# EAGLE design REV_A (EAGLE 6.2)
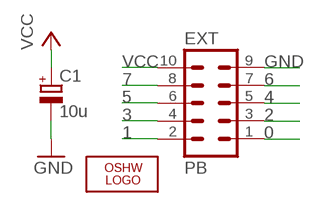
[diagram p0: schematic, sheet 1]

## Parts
C1  10u  CPOL-EUSMCA  [SMC_A]
EXT  PB  ML10  [ML10]
LOGO1  OSHW_LOGO_8MIL  [OSHW_8X150_NOTEXT_MASK]

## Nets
0: EXT.1
1: EXT.2
2: EXT.3
3: EXT.4
4: EXT.5
5: EXT.6
6: EXT.7
7: EXT.8
GND: C1.- EXT.9
VCC: C1.+ EXT.10

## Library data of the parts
C1 = rcl:CPOL-EU: POLARIZED CAPACITOR, European symbol
EXT = con-harting-ml2:ML10: HARTING; OC_FARNELL: unknown; OC_NEWARK: unknown
LOGO1 = ohw-logo:OSHW_LOGO_8MIL

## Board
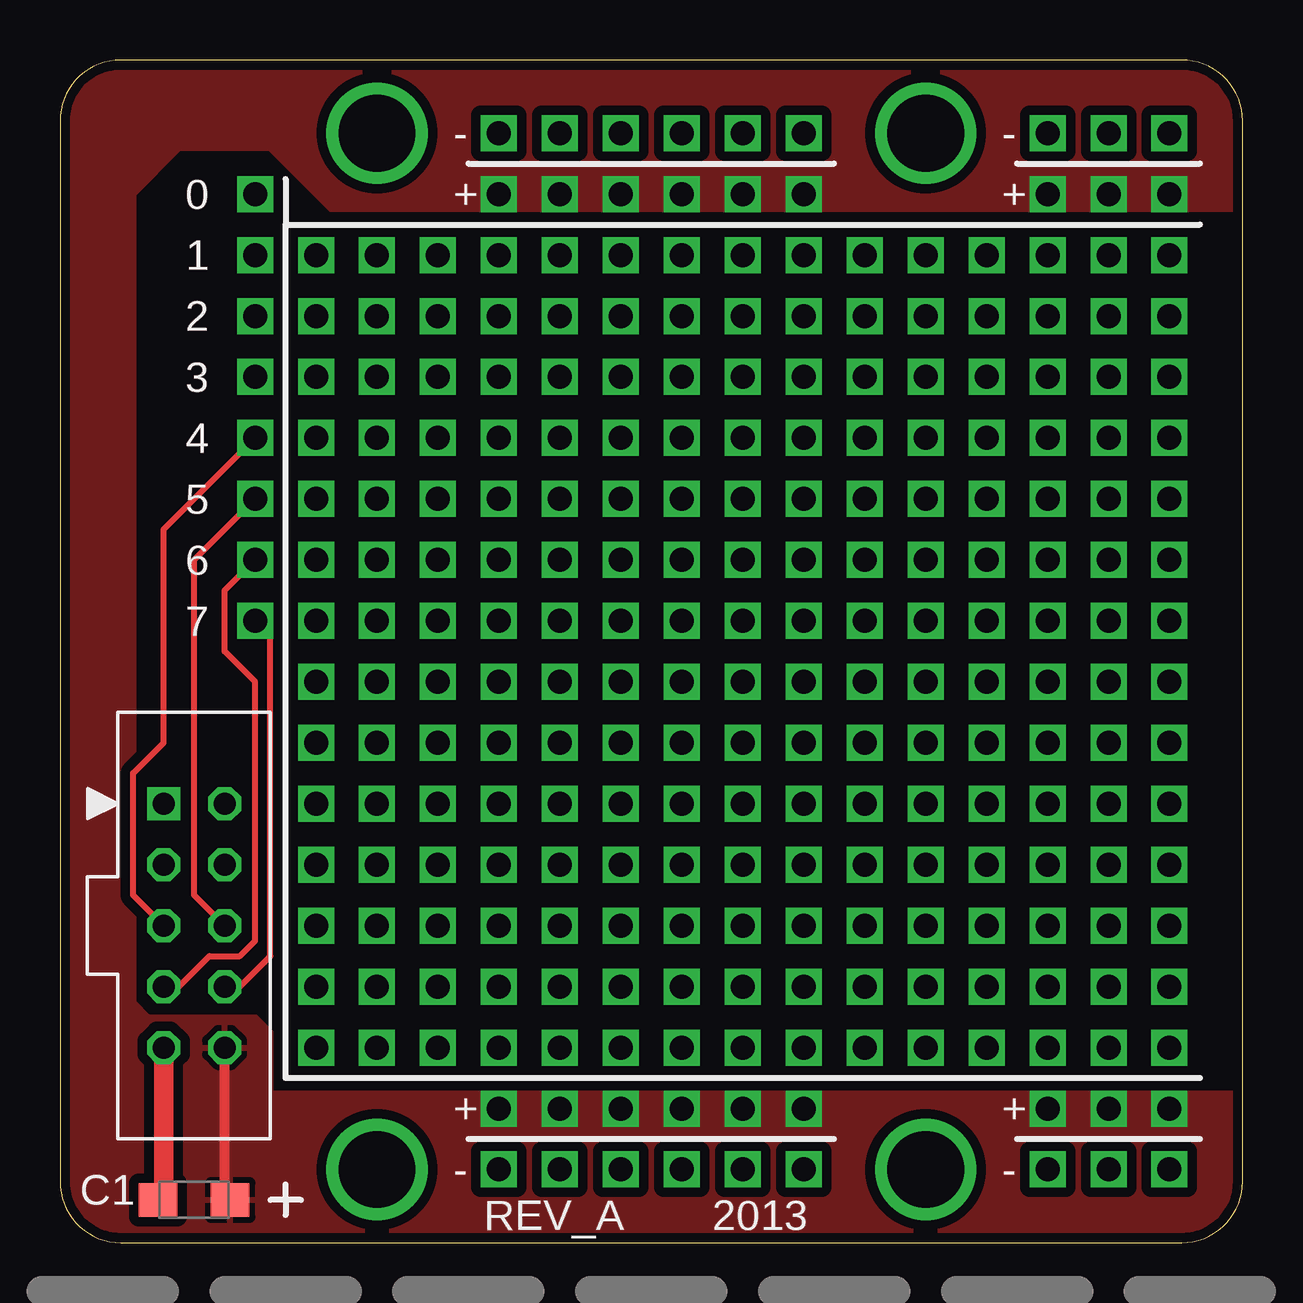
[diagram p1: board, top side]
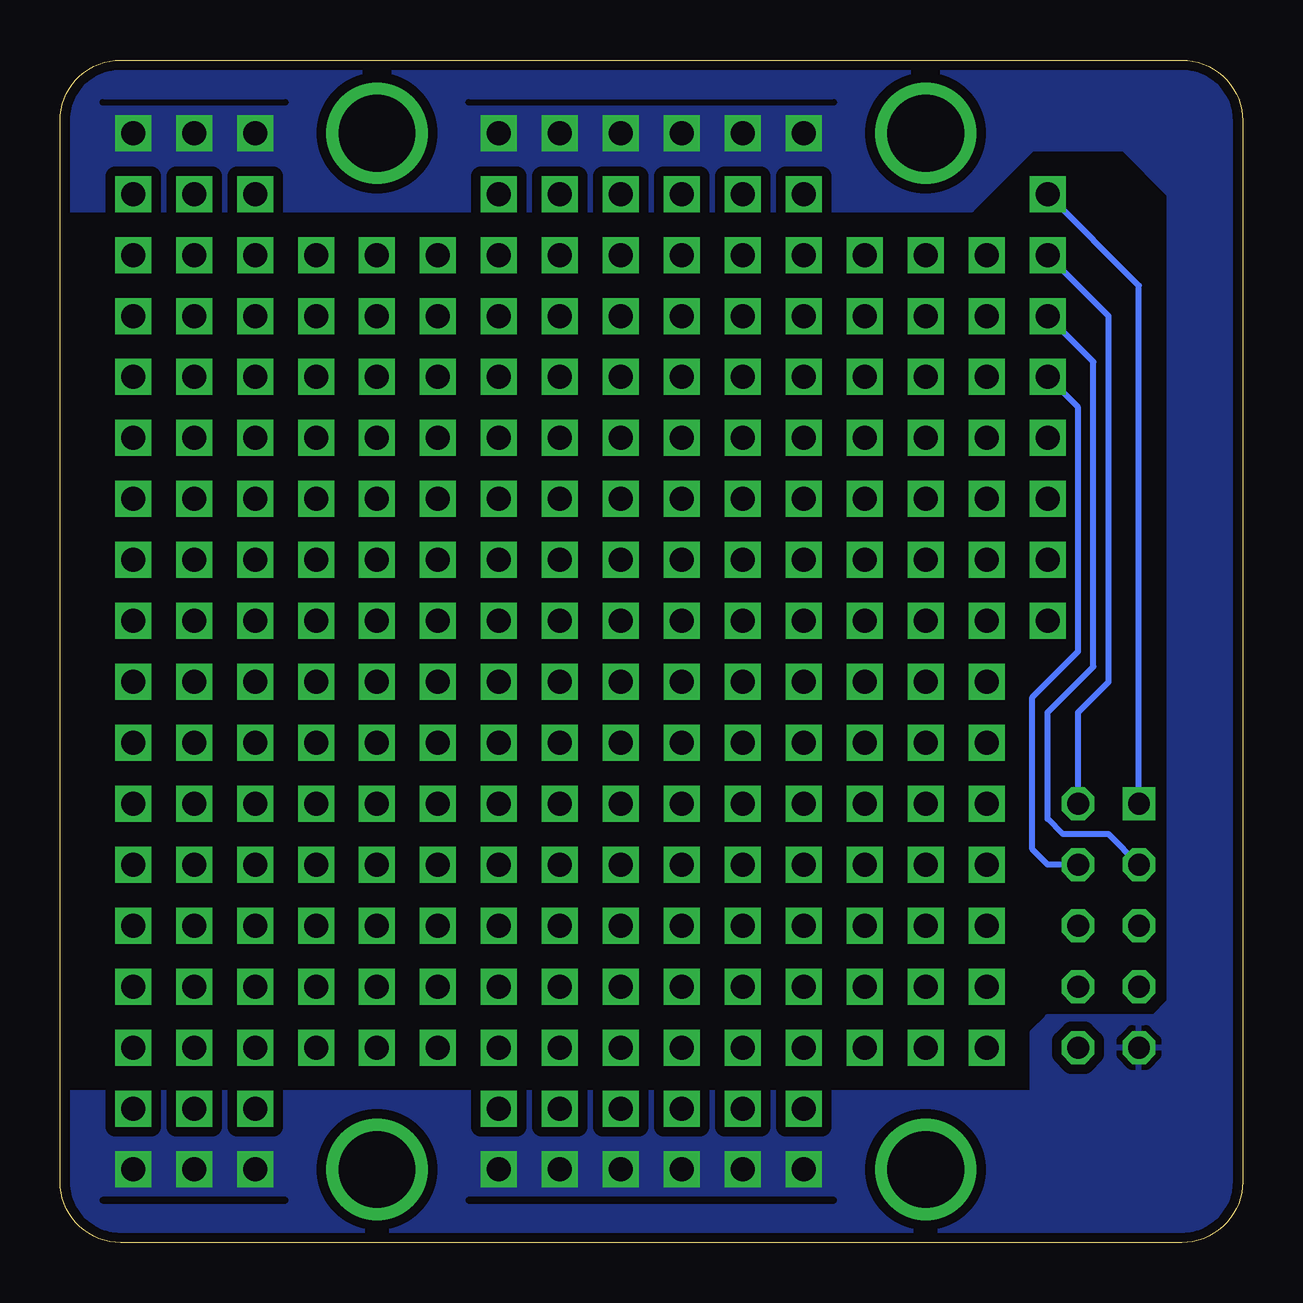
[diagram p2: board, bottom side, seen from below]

Size 49.28 x 49.28 mm. Coordinates in mm from the lower left corner, seen from the top.
Outline: 46.74,49.28 2.54,49.28 arc90 0,46.74 0,2.54 arc90 2.54,0 46.74,0 arc90 49.28,2.54 49.28,46.74 arc90 46.74,49.28
Copper layers (1*2*15*16): Top 0.035mm / dielectric 0.2mm / layer 2 0.0175mm / dielectric 1.1mm / layer 15 0.0175mm / dielectric 0.2mm / Bottom 0.035mm
Design rules: minimum track width 6mil, minimum drill 12mil, track to track 6mil, track to pad 6mil, pad to pad 6mil, via to via 6mil, smd to smd 0mil, copper to edge 10mil, drill to drill 10mil, minimum pad ring 6mil, minimum via ring 6mil, stop-mask expansion 2mil, vias tented up to drill 25mil, thermal gap 10mil

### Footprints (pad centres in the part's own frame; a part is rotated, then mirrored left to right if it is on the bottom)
SMC_A = smd 1.6 x 1.4: + -1.5,0; - 1.5,0
ML10 = drill 0.914 square: 1 -5.08,-1.27 | drill 0.914 octagon: 2 -5.08,1.27; 3 -2.54,-1.27; 4 -2.54,1.27; 5 0,-1.27; 6 0,1.27; 7 2.54,-1.27; 8 2.54,1.27; 9 5.08,-1.27; 10 5.08,1.27

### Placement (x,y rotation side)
C1  5.59,1.78 180 top
EXT  5.59,13.21 270 top
LOGO1  5.59,46.86 315 bottom

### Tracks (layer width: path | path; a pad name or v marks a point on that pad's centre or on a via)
0  (via drill 1)
  Bottom 0.254: EXT.1 4.32,39.88 v8.13,43.69
1  (via drill 1)
  Bottom 0.254: EXT.2 6.86,22.1 5.59,23.37 5.59,38.61 v8.13,41.15
2  (via drill 1)
  Bottom 0.254: EXT.3 5.59,17.02 7.49,17.02 8.13,17.65 8.13,22.1 6.22,24 6.22,36.7 v8.13,38.61
3  (via drill 1)
  Bottom 0.254: v8.13,36.07 6.86,34.8 6.86,24.64 8.76,22.73 8.76,16.38 8.13,15.75 EXT.4
4  (via drill 1)
  Top 0.254: EXT.5 3.05,14.48 3.05,19.56 4.32,20.83 4.32,29.72 v8.13,33.53
5  (via drill 1)
  Top 0.254: EXT.6 5.59,14.48 5.59,28.45 v8.13,30.99
6  (via drill 1)
  Top 0.254: EXT.7 4.95,10.67 6.22,11.94 7.49,11.94 8.13,12.57 8.13,23.37 6.86,24.64 6.86,27.18 v8.13,28.45
7  (via drill 1)
  Top 0.254: EXT.8 7.49,10.67 8.76,11.94 8.76,25.27 v8.13,25.91
GND  (via drill 1)
  Top 0.406: C1.- 4.32,1.78
  Top 0.813: 4.32,1.78 EXT.9
  other vias: 18.29,3.05 20.83,3.05 23.37,3.05 25.91,3.05 28.45,3.05 30.99,3.05 41.15,3.05 43.69,3.05 46.23,3.05 18.29,46.23 20.83,46.23 23.37,46.23 25.91,46.23 28.45,46.23 30.99,46.23 41.15,46.23 43.69,46.23 46.23,46.23
  pour Bottom (isolate 0.406): 50.04,6.22 50.04,-0.76 -0.76,-0.76 -0.76,49.4 47.5,49.4 50.04,46.86 50.04,43.05 11.3,43.05 8.76,45.59 4.95,45.59 3.05,43.69 3.05,10.03 3.68,9.4 8.13,9.4 8.76,8.76 8.76,6.22
N$3  (via drill 3.2)
  other vias: 13.21,46.23
N$4  (via drill 1)
  other vias: 10.67,41.15
N$5  (via drill 1)
  other vias: 13.21,41.15
N$6  (via drill 1)
  other vias: 15.75,41.15
N$7  (via drill 1)
  other vias: 18.29,41.15
N$8  (via drill 1)
  other vias: 20.83,41.15
N$9  (via drill 1)
  other vias: 23.37,41.15
N$10  (via drill 1)
  other vias: 25.91,41.15
N$11  (via drill 1)
  other vias: 28.45,41.15
N$12  (via drill 1)
  other vias: 30.99,41.15
N$13  (via drill 1)
  other vias: 33.53,41.15
N$14  (via drill 1)
  other vias: 36.07,41.15
N$15  (via drill 1)
  other vias: 38.61,41.15
N$16  (via drill 1)
  other vias: 41.15,41.15
N$17  (via drill 1)
  other vias: 43.69,41.15
N$18  (via drill 1)
  other vias: 46.23,41.15
N$21  (via drill 3.2)
  other vias: 36.07,46.23
N$22  (via drill 1)
  other vias: 10.67,38.61
N$23  (via drill 1)
  other vias: 13.21,38.61
N$24  (via drill 1)
  other vias: 15.75,38.61
N$25  (via drill 1)
  other vias: 18.29,38.61
N$26  (via drill 1)
  other vias: 20.83,38.61
N$27  (via drill 1)
  other vias: 23.37,38.61
N$28  (via drill 1)
  other vias: 25.91,38.61
N$29  (via drill 1)
  other vias: 28.45,38.61
N$30  (via drill 1)
  other vias: 30.99,38.61
N$31  (via drill 1)
  other vias: 33.53,38.61
N$32  (via drill 1)
  other vias: 36.07,38.61
N$33  (via drill 1)
  other vias: 38.61,38.61
N$34  (via drill 1)
  other vias: 41.15,38.61
N$35  (via drill 1)
  other vias: 43.69,38.61
N$36  (via drill 1)
  other vias: 46.23,38.61
N$39
  cutout Bottom: 17.02,1.78 32.26,1.78 32.26,1.75 17.02,1.75
N$40  (via drill 1)
  other vias: 10.67,36.07
N$41  (via drill 1)
  other vias: 13.21,36.07
N$42  (via drill 1)
  other vias: 15.75,36.07
N$43  (via drill 1)
  other vias: 18.29,36.07
N$44  (via drill 1)
  other vias: 20.83,36.07
N$45  (via drill 1)
  other vias: 23.37,36.07
N$46  (via drill 1)
  other vias: 25.91,36.07
N$47  (via drill 1)
  other vias: 28.45,36.07
N$48  (via drill 1)
  other vias: 30.99,36.07
N$49  (via drill 1)
  other vias: 33.53,36.07
N$50  (via drill 1)
  other vias: 36.07,36.07
N$51  (via drill 1)
  other vias: 38.61,36.07
N$52  (via drill 1)
  other vias: 41.15,36.07
N$53  (via drill 1)
  other vias: 43.69,36.07
N$54  (via drill 1)
  other vias: 46.23,36.07
N$57
  cutout Bottom: 39.88,1.78 47.5,1.78 47.5,1.75 39.88,1.75
N$58  (via drill 1)
  other vias: 10.67,33.53
N$59  (via drill 1)
  other vias: 13.21,33.53
N$60  (via drill 1)
  other vias: 15.75,33.53
N$61  (via drill 1)
  other vias: 18.29,33.53
N$62  (via drill 1)
  other vias: 20.83,33.53
N$63  (via drill 1)
  other vias: 23.37,33.53
N$64  (via drill 1)
  other vias: 25.91,33.53
N$65  (via drill 1)
  other vias: 28.45,33.53
N$66  (via drill 1)
  other vias: 30.99,33.53
N$67  (via drill 1)
  other vias: 33.53,33.53
N$68  (via drill 1)
  other vias: 36.07,33.53
N$69  (via drill 1)
  other vias: 38.61,33.53
N$70  (via drill 1)
  other vias: 41.15,33.53
N$71  (via drill 1)
  other vias: 43.69,33.53
N$72  (via drill 1)
  other vias: 46.23,33.53
N$73
  cutout Bottom: 17.02,47.5 32.26,47.5 32.26,47.52 17.02,47.52
N$74
  cutout Bottom: 39.88,47.5 47.5,47.5 47.5,47.52 39.88,47.52
N$76  (via drill 1)
  other vias: 10.67,30.99
N$77  (via drill 1)
  other vias: 13.21,30.99
N$78  (via drill 1)
  other vias: 15.75,30.99
N$79  (via drill 1)
  other vias: 18.29,30.99
N$80  (via drill 1)
  other vias: 20.83,30.99
N$81  (via drill 1)
  other vias: 23.37,30.99
N$82  (via drill 1)
  other vias: 25.91,30.99
N$83  (via drill 1)
  other vias: 28.45,30.99
N$84  (via drill 1)
  other vias: 30.99,30.99
N$85  (via drill 1)
  other vias: 33.53,30.99
N$86  (via drill 1)
  other vias: 36.07,30.99
N$87  (via drill 1)
  other vias: 38.61,30.99
N$88  (via drill 1)
  other vias: 41.15,30.99
N$89  (via drill 1)
  other vias: 43.69,30.99
N$90  (via drill 1)
  other vias: 46.23,30.99
N$93  (via drill 1)
  other vias: 10.67,28.45
N$94  (via drill 1)
  other vias: 13.21,28.45
N$95  (via drill 1)
  other vias: 15.75,28.45
N$96  (via drill 1)
  other vias: 18.29,28.45
N$97  (via drill 1)
  other vias: 20.83,28.45
N$98  (via drill 1)
  other vias: 23.37,28.45
N$99  (via drill 1)
  other vias: 25.91,28.45
N$100  (via drill 1)
  other vias: 28.45,28.45
N$101  (via drill 1)
  other vias: 30.99,28.45
N$102  (via drill 1)
  other vias: 33.53,28.45
N$103  (via drill 1)
  other vias: 36.07,28.45
N$104  (via drill 1)
  other vias: 38.61,28.45
N$105  (via drill 1)
  other vias: 41.15,28.45
N$106  (via drill 1)
  other vias: 43.69,28.45
N$107  (via drill 1)
  other vias: 46.23,28.45
N$111  (via drill 1)
  other vias: 10.67,25.91
N$112  (via drill 1)
  other vias: 13.21,25.91
N$113  (via drill 1)
  other vias: 15.75,25.91
N$114  (via drill 1)
  other vias: 18.29,25.91
N$115  (via drill 1)
  other vias: 20.83,25.91
N$116  (via drill 1)
  other vias: 23.37,25.91
N$117  (via drill 1)
  other vias: 25.91,25.91
N$118  (via drill 1)
  other vias: 28.45,25.91
N$119  (via drill 1)
  other vias: 30.99,25.91
N$120  (via drill 1)
  other vias: 33.53,25.91
N$121  (via drill 1)
  other vias: 36.07,25.91
N$122  (via drill 1)
  other vias: 38.61,25.91
N$123  (via drill 1)
  other vias: 41.15,25.91
N$124  (via drill 1)
  other vias: 43.69,25.91
N$125  (via drill 1)
  other vias: 46.23,25.91
N$128  (via drill 3.2)
  other vias: 36.07,3.05
N$129  (via drill 1)
  other vias: 10.67,23.37
N$130  (via drill 1)
  other vias: 13.21,23.37
N$131  (via drill 1)
  other vias: 15.75,23.37
N$132  (via drill 1)
  other vias: 18.29,23.37
N$133  (via drill 1)
  other vias: 20.83,23.37
N$134  (via drill 1)
  other vias: 23.37,23.37
N$135  (via drill 1)
  other vias: 25.91,23.37
N$136  (via drill 1)
  other vias: 28.45,23.37
N$137  (via drill 1)
  other vias: 30.99,23.37
N$138  (via drill 1)
  other vias: 33.53,23.37
N$139  (via drill 1)
  other vias: 36.07,23.37
N$140  (via drill 1)
  other vias: 38.61,23.37
N$141  (via drill 1)
  other vias: 41.15,23.37
N$142  (via drill 1)
  other vias: 43.69,23.37
N$143  (via drill 1)
  other vias: 46.23,23.37
N$144  (via drill 3.2)
  other vias: 13.21,3.05
N$183  (via drill 1)
  other vias: 10.67,20.83
N$184  (via drill 1)
  other vias: 13.21,20.83
N$185  (via drill 1)
  other vias: 15.75,20.83
N$186  (via drill 1)
  other vias: 18.29,20.83
N$187  (via drill 1)
  other vias: 20.83,20.83
N$188  (via drill 1)
  other vias: 23.37,20.83
N$189  (via drill 1)
  other vias: 25.91,20.83
N$190  (via drill 1)
  other vias: 28.45,20.83
N$191  (via drill 1)
  other vias: 30.99,20.83
N$192  (via drill 1)
  other vias: 33.53,20.83
N$193  (via drill 1)
  other vias: 36.07,20.83
N$194  (via drill 1)
  other vias: 38.61,20.83
N$195  (via drill 1)
  other vias: 41.15,20.83
N$196  (via drill 1)
  other vias: 43.69,20.83
N$197  (via drill 1)
  other vias: 46.23,20.83
N$198  (via drill 1)
  other vias: 10.67,18.29
N$199  (via drill 1)
  other vias: 13.21,18.29
N$200  (via drill 1)
  other vias: 15.75,18.29
N$201  (via drill 1)
  other vias: 18.29,18.29
N$202  (via drill 1)
  other vias: 20.83,18.29
N$203  (via drill 1)
  other vias: 23.37,18.29
N$204  (via drill 1)
  other vias: 25.91,18.29
N$205  (via drill 1)
  other vias: 28.45,18.29
N$206  (via drill 1)
  other vias: 30.99,18.29
N$207  (via drill 1)
  other vias: 33.53,18.29
N$208  (via drill 1)
  other vias: 36.07,18.29
N$209  (via drill 1)
  other vias: 38.61,18.29
N$210  (via drill 1)
  other vias: 41.15,18.29
N$211  (via drill 1)
  other vias: 43.69,18.29
N$212  (via drill 1)
  other vias: 46.23,18.29
N$213  (via drill 1)
  other vias: 10.67,15.75
N$214  (via drill 1)
  other vias: 13.21,15.75
N$215  (via drill 1)
  other vias: 15.75,15.75
N$216  (via drill 1)
  other vias: 18.29,15.75
N$217  (via drill 1)
  other vias: 20.83,15.75
N$218  (via drill 1)
  other vias: 23.37,15.75
N$219  (via drill 1)
  other vias: 25.91,15.75
N$220  (via drill 1)
  other vias: 28.45,15.75
N$221  (via drill 1)
  other vias: 30.99,15.75
N$222  (via drill 1)
  other vias: 33.53,15.75
N$223  (via drill 1)
  other vias: 36.07,15.75
N$224  (via drill 1)
  other vias: 38.61,15.75
N$225  (via drill 1)
  other vias: 41.15,15.75
N$226  (via drill 1)
  other vias: 43.69,15.75
N$227  (via drill 1)
  other vias: 46.23,15.75
N$228  (via drill 1)
  other vias: 10.67,13.21
N$229  (via drill 1)
  other vias: 13.21,13.21
N$230  (via drill 1)
  other vias: 15.75,13.21
N$231  (via drill 1)
  other vias: 18.29,13.21
N$232  (via drill 1)
  other vias: 20.83,13.21
N$233  (via drill 1)
  other vias: 23.37,13.21
N$234  (via drill 1)
  other vias: 25.91,13.21
N$235  (via drill 1)
  other vias: 28.45,13.21
N$236  (via drill 1)
  other vias: 30.99,13.21
N$237  (via drill 1)
  other vias: 33.53,13.21
N$238  (via drill 1)
  other vias: 36.07,13.21
N$239  (via drill 1)
  other vias: 38.61,13.21
N$240  (via drill 1)
  other vias: 41.15,13.21
N$241  (via drill 1)
  other vias: 43.69,13.21
N$242  (via drill 1)
  other vias: 46.23,13.21
N$243  (via drill 1)
  other vias: 10.67,10.67
N$244  (via drill 1)
  other vias: 13.21,10.67
N$245  (via drill 1)
  other vias: 15.75,10.67
N$246  (via drill 1)
  other vias: 18.29,10.67
N$247  (via drill 1)
  other vias: 20.83,10.67
N$248  (via drill 1)
  other vias: 23.37,10.67
N$249  (via drill 1)
  other vias: 25.91,10.67
N$250  (via drill 1)
  other vias: 28.45,10.67
N$251  (via drill 1)
  other vias: 30.99,10.67
N$252  (via drill 1)
  other vias: 33.53,10.67
N$253  (via drill 1)
  other vias: 36.07,10.67
N$254  (via drill 1)
  other vias: 38.61,10.67
N$255  (via drill 1)
  other vias: 41.15,10.67
N$256  (via drill 1)
  other vias: 43.69,10.67
N$257  (via drill 1)
  other vias: 46.23,10.67
N$258  (via drill 1)
  other vias: 10.67,8.13
N$259  (via drill 1)
  other vias: 13.21,8.13
N$260  (via drill 1)
  other vias: 15.75,8.13
N$261  (via drill 1)
  other vias: 18.29,8.13
N$262  (via drill 1)
  other vias: 20.83,8.13
N$263  (via drill 1)
  other vias: 23.37,8.13
N$264  (via drill 1)
  other vias: 25.91,8.13
N$265  (via drill 1)
  other vias: 28.45,8.13
N$266  (via drill 1)
  other vias: 30.99,8.13
N$267  (via drill 1)
  other vias: 33.53,8.13
N$268  (via drill 1)
  other vias: 36.07,8.13
N$269  (via drill 1)
  other vias: 38.61,8.13
N$270  (via drill 1)
  other vias: 41.15,8.13
N$271  (via drill 1)
  other vias: 43.69,8.13
N$272  (via drill 1)
  other vias: 46.23,8.13
VCC  (via drill 1)
  Top 0.406: C1.+ 6.86,1.78 EXT.10
  other vias: 18.29,5.59 20.83,5.59 23.37,5.59 25.91,5.59 28.45,5.59 30.99,5.59 41.15,5.59 43.69,5.59 46.23,5.59 18.29,43.69 20.83,43.69 23.37,43.69 25.91,43.69 28.45,43.69 30.99,43.69 41.15,43.69 43.69,43.69 46.23,43.69
  pour Top (isolate 0.406): 50.04,6.22 50.04,-0.76 -0.76,-0.76 -0.76,49.4 47.5,49.4 50.04,46.86 50.04,43.05 11.3,43.05 8.76,45.59 4.95,45.59 3.05,43.69 3.05,10.03 3.68,9.4 8.13,9.4 8.76,8.76 8.76,6.22

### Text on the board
tPlace: - | - | 0 | + | + | 1 | 2 | 3 | 4 | 5 | 6 | 7 | + | + | - | -
tNames: 2013
tValues: 1 | 1 | 1 | 1
bStop: slashhome.se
